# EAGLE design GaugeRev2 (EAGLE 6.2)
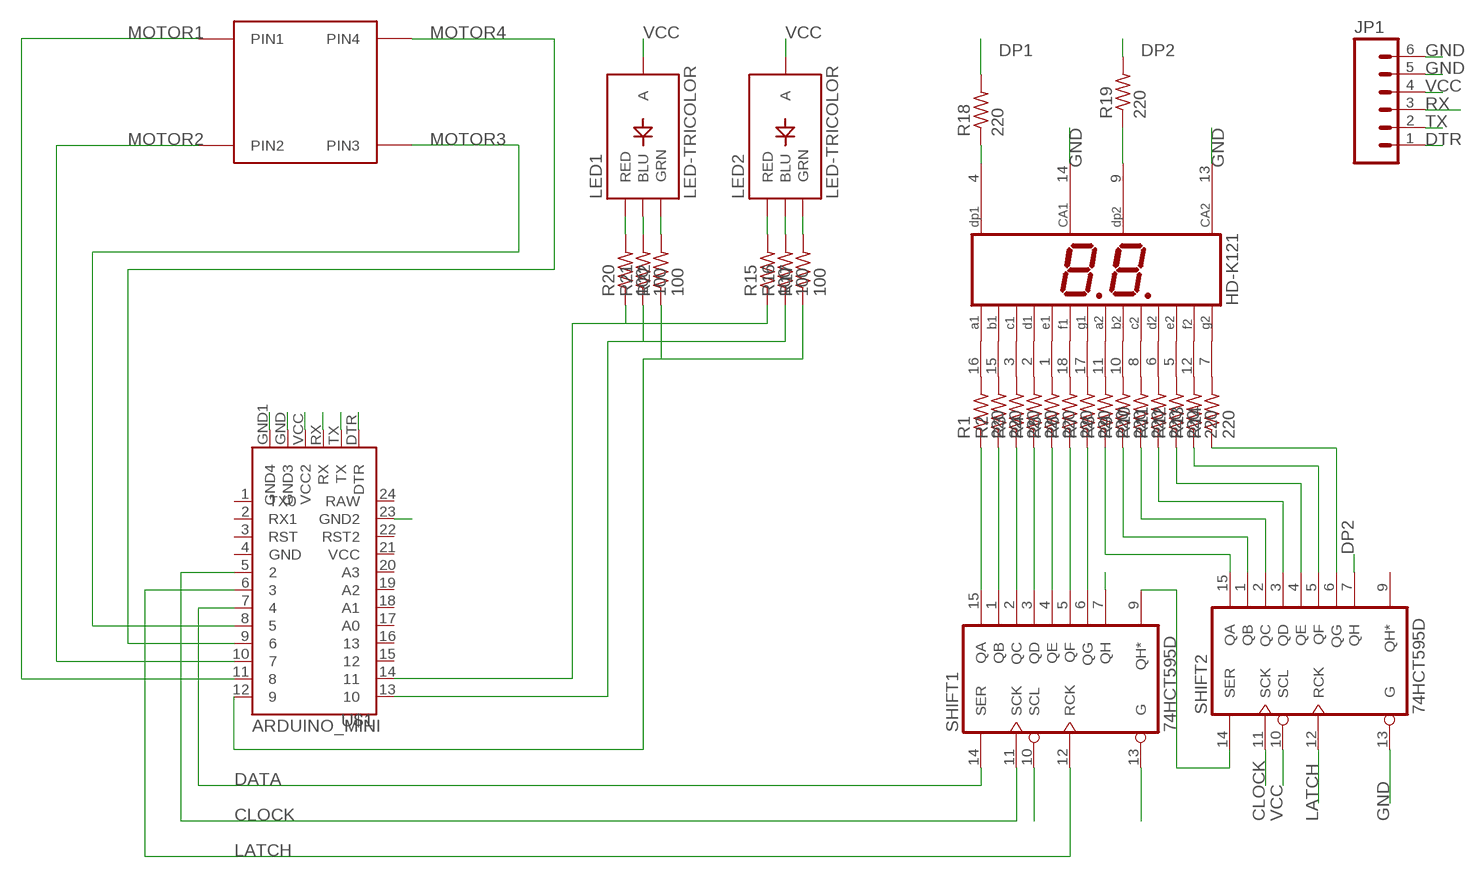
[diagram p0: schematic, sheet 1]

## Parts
DIS2  HD-K121  [HDSP-R]
JP1  M06SIP  [1X06]
LED1  LED-TRICOLOR  [LED-TRICOLOR-SMD]
LED2  LED-TRICOLOR  [LED-TRICOLOR-SMD]
R1  220  R-US_R1206  [R1206]
R2  220  R-US_R1206  [R1206]
R3  220  R-US_R1206  [R1206]
R4  220  R-US_R1206  [R1206]
R5  220  R-US_R1206  [R1206]
R6  220  R-US_R1206  [R1206]
R7  220  R-US_R1206  [R1206]
R8  220  R-US_R1206  [R1206]
R9  220  R-US_R1206  [R1206]
R10  220  R-US_R1206  [R1206]
R11  220  R-US_R1206  [R1206]
R12  220  R-US_R1206  [R1206]
R13  220  R-US_R1206  [R1206]
R14  220  R-US_R1206  [R1206]
R15  100  R-US_R1206  [R1206]
R16  100  R-US_R1206  [R1206]
R17  100  R-US_R1206  [R1206]
R18  220  R-US_R1206  [R1206]
R19  220  R-US_R1206  [R1206]
R20  100  R-US_R1206  [R1206]
R21  100  R-US_R1206  [R1206]
R22  100  R-US_R1206  [R1206]
SHIFT1  74HCT595D  [SO16]
SHIFT2  74HCT595D  [SO16]
U$1  ARDUINO_MINI  [ARDUINO_MINI]
U$4  VID29  [VID29]

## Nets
1: DIS2.4(DP1) R18.1
2: DIS2.9(DP2) R19.1
A1: R1.1 SHIFT1.15(QA)
A2: R8.1 SHIFT2.15(QA)
B1: R2.1 SHIFT1.1(QB)
B2: R9.1 SHIFT2.1(QB)
C1: R3.1 SHIFT1.2(QC)
CLOCK: SHIFT1.11(SCK) SHIFT2.11(SCK) U$1.5
D1: R4.1 SHIFT1.3(QD)
DATA: SHIFT1.14(SER) U$1.7
DP1: R18.2 SHIFT1.7(QH)
DP2: R19.2 SHIFT2.7(QH)
DTR: JP1.1 U$1.DTR
E1: R5.1 SHIFT1.4(QE)
F1: R6.1 SHIFT1.5(QF)
G1: R7.1 SHIFT1.6(QG)
G2: R14.1 SHIFT2.6(QG)
GND: DIS2.13(CA2) DIS2.14(CA1) JP1.5 JP1.6 SHIFT1.13(G) SHIFT2.13(G) U$1.23(GND2) U$1.GND1(GND4) U$1.GND(GND3)
LATCH: SHIFT1.12(RCK) SHIFT2.12(RCK) U$1.6
LED_B: R16.1 R21.1 U$1.13
LED_G: R15.1 R20.1 U$1.14
LED_R: R17.1 R22.1 U$1.12
MOTOR1: U$1.11 U$4.PIN1
MOTOR2: U$1.10 U$4.PIN2
MOTOR3: U$1.8 U$4.PIN3
MOTOR4: U$1.9 U$4.PIN4
N$1: DIS2.16(A1) R1.2
N$2: DIS2.15(B1) R2.2
N$3: DIS2.3(C1) R3.2
N$4: DIS2.2(D1) R4.2
N$5: DIS2.1(E1) R5.2
N$6: DIS2.18(F1) R6.2
N$7: DIS2.17(G1) R7.2
N$8: DIS2.11(A2) R8.2
N$9: DIS2.10(B2) R9.2
N$10: DIS2.8(C2) R10.2
N$11: DIS2.6(D2) R11.2
N$12: DIS2.5(E2) R12.2
N$13: DIS2.12(F2) R13.2
N$14: DIS2.7(G2) R14.2
N$15: LED2.G(GRN) R17.2
N$16: LED2.B(BLU) R16.2
N$19: R10.1 SHIFT2.2(QC)
N$20: R11.1 SHIFT2.3(QD)
N$21: R12.1 SHIFT2.4(QE)
N$22: R13.1 SHIFT2.5(QF)
N$23: LED2.R(RED) R15.2
N$24: LED1.G(GRN) R22.2
N$25: LED1.B(BLU) R21.2
N$26: LED1.R(RED) R20.2
Q*: SHIFT1.9(QH*) SHIFT2.14(SER)
RX: JP1.3 U$1.RX
TX: JP1.2 U$1.TX
VCC: JP1.4 LED1.A LED2.A SHIFT1.10(SCL) SHIFT2.10(SCL) U$1.VCC(VCC2)
Unconnected: SHIFT2.9(QH*) U$1.1(TX0) U$1.2(RX1) U$1.3(RST) U$1.4(GND) U$1.15 U$1.16 U$1.17(A0) U$1.18(A1) U$1.19(A2) U$1.20(A3) U$1.21(VCC) U$1.22(RST2) U$1.24(RAW)

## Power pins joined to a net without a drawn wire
GND: SHIFT1.8(GND) SHIFT2.8(GND)
VCC: SHIFT1.16(VCC) SHIFT2.16(VCC)

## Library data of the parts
DIS2 = HDSP-523E:HD-K121: LED DISPLAY 2 x 1 character 7 segment, decimal points right; OC_FARNELL: unknown; OC_NEWARK: unknown
JP1 = SparkFun:M06: Header 6 Standard 6-pin 0.1" header. Use with straight break away headers (SKU : PRT-00116), right angle break away headers (PRT-00553), swiss pins (PRT-00743), machine pins (PRT-00117), and female headers (PRT-00115). Molex polarized connector foot print use with SKU : PRT-08094 with associated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
LED1 LED2 = SparkFun:LED-TRICOLOR: Tri-Color LED SMD Proven layout and schematic for triple color LED in SMD package - common anode. Spark Fun Electronics SKU : COM-07844
R1-R22 = resistor:R-US_: RESISTOR, American symbol
SHIFT1 SHIFT2 = 74xx-eu:74*595: 8-bit SHIFT REGISTER, output latch
U$1 = SparkFun:ARDUINO_MINI
U$4 = Evans:VID29

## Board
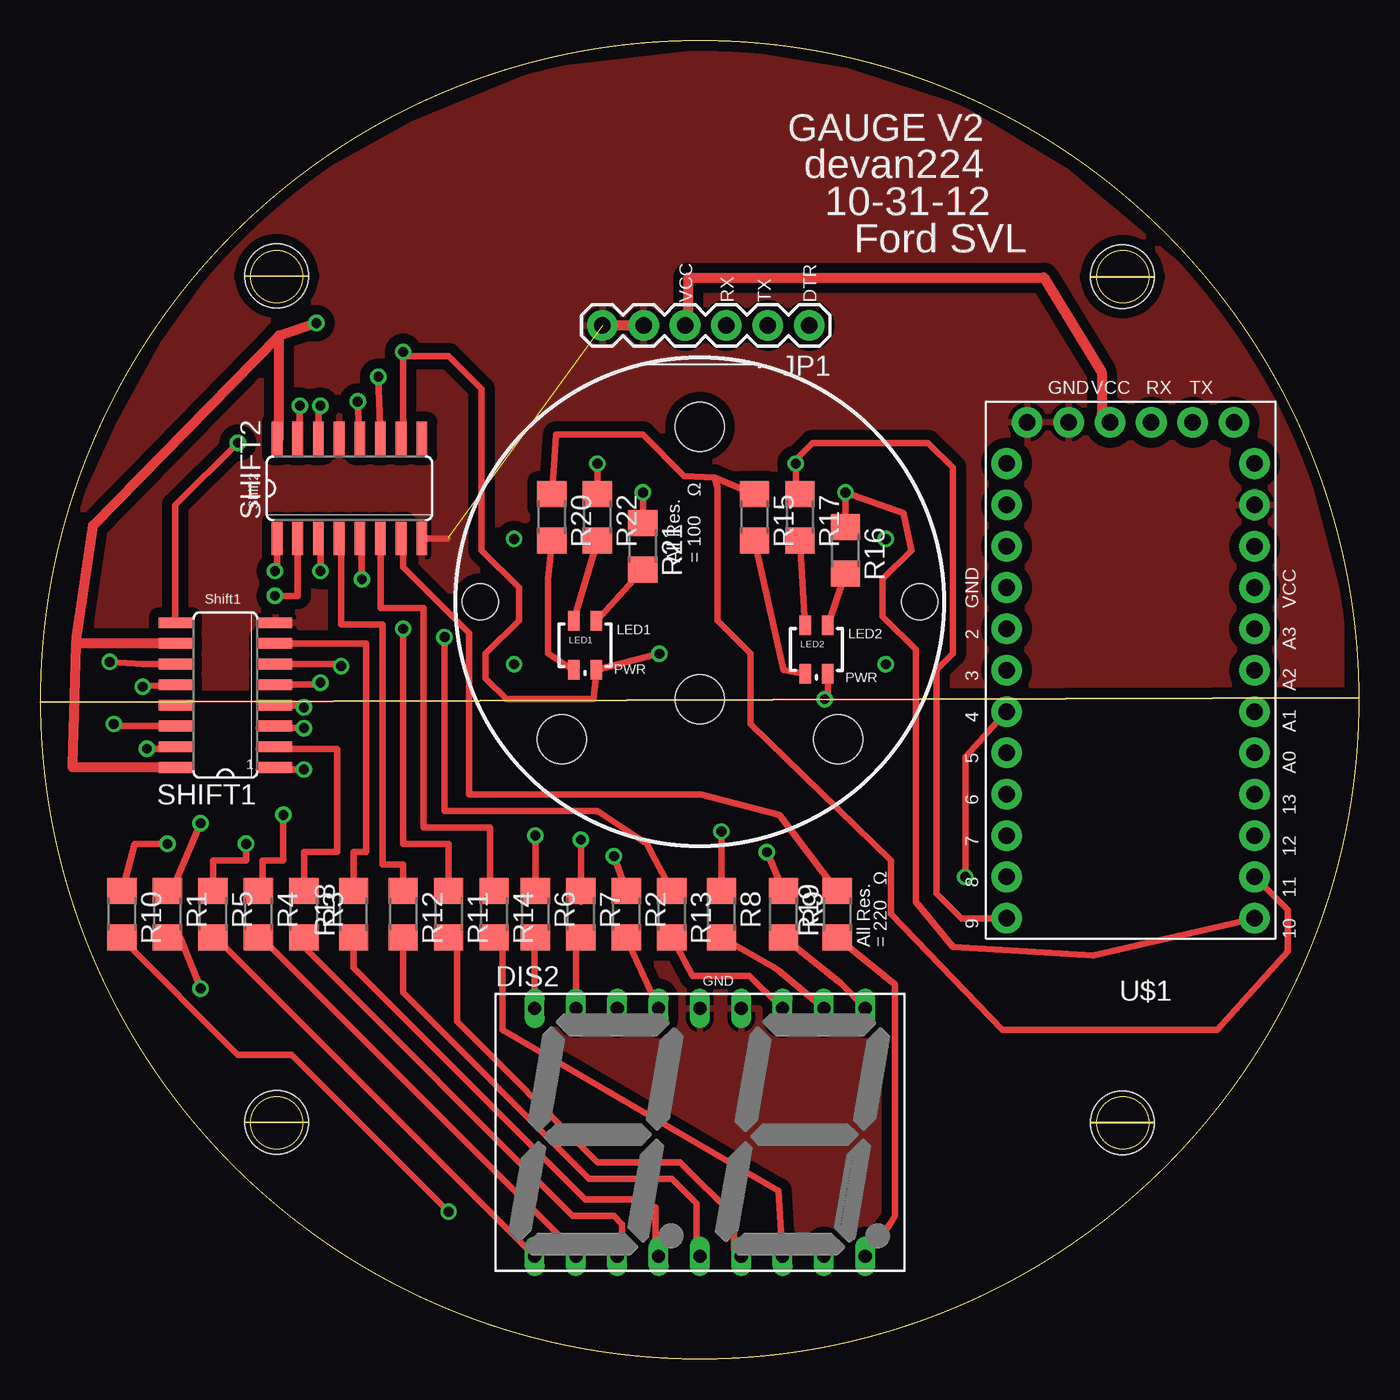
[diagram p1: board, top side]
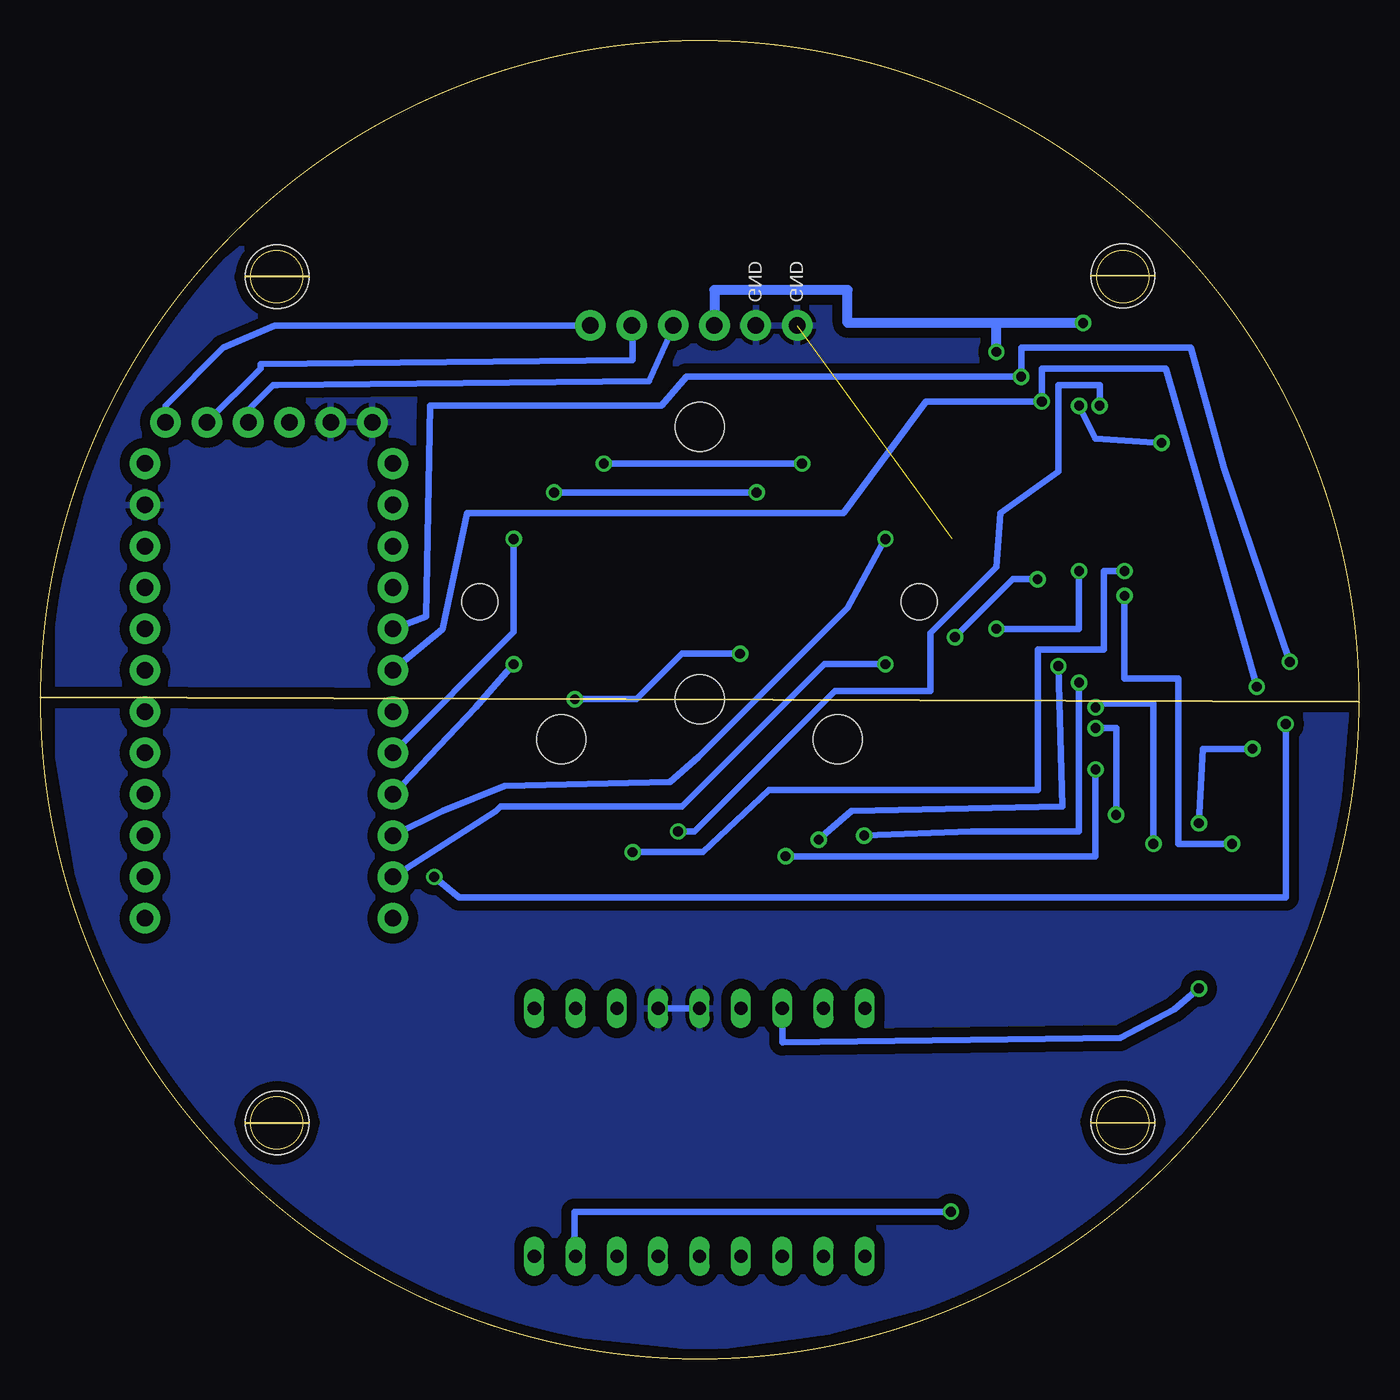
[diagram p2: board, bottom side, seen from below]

Size 81 x 81 mm. Coordinates in mm from the lower left corner, seen from the top.
Outline: circle at 66.5,66.5 radius 1.6
Outline: circle at 14.5,66.5 radius 1.6
Outline: circle at 66.5,14.5 radius 1.6
Outline: circle at 14.5,14.5 radius 1.6
Outline: circle at 40.5,40.5 radius 40.5
Copper layers (1*16): Top 0.0178mm / dielectric 59mil / Bottom 0.0178mm
Design rules: minimum track width 6mil, minimum drill 14mil, track to track 6mil, track to pad 6mil, pad to pad 6mil, via to via 6mil, smd to smd 6mil, copper to edge 20mil, drill to drill 16mil, minimum pad ring 8mil, minimum via ring 8mil, stop-mask expansion 3mil, vias tented up to drill 0mil, thermal gap 10mil
Holes 3.9 mm at 14.5,66.55 66.47,66.5 66.47,14.5 14.5,14.53

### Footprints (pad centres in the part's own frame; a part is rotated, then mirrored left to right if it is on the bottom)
HDSP-R = drill 0.813 long: 1 -10.16,-7.62; 2 -7.62,-7.62; 3 -5.08,-7.62; 4 -2.54,-7.62; 5 0,-7.62; 6 2.54,-7.62; 7 5.08,-7.62; 8 7.62,-7.62; 9 10.16,-7.62; 10 10.16,7.62; 11 7.62,7.62; 12 5.08,7.62; 13 2.54,7.62; 14 0,7.62; 15 -2.54,7.62; 16 -5.08,7.62; 17 -7.62,7.62; 18 -10.16,7.62
1X06 = drill 1.016 pad 1.88: 1 0,0; 2 2.54,0; 3 5.08,0; 4 7.62,0; 5 10.16,0; 6 12.7,0
LED-TRICOLOR-SMD = smd 0.7 x 1.2: A 0.7,-1.5; B 0.7,1.5; G -0.7,1.5; R -0.7,-1.5
R1206 = smd 1.6 x 1.803: 1 -1.422,0; 2 1.422,0
SO16 = smd 0.66 x 2.032: 1 -4.445,-3.073; 2 -3.175,-3.073; 3 -1.905,-3.073; 4 -0.635,-3.073; 5 0.635,-3.073; 6 1.905,-3.073; 7 3.175,-3.073; 8 4.445,-3.073; 9 4.445,3.073; 10 3.175,3.073; 11 1.905,3.073; 12 0.635,3.073; 13 -0.635,3.073; 14 -1.905,3.073; 15 -3.175,3.073; 16 -4.445,3.073
ARDUINO_MINI = drill 1.016 pad 1.88: 1 -7.62,12.7; 2 -7.62,10.16; 3 -7.62,7.62; 4 -7.62,5.08; 5 -7.62,2.54; 6 -7.62,0; 7 -7.62,-2.54; 8 -7.62,-5.08; 9 -7.62,-7.62; 10 -7.62,-10.16; 11 -7.62,-12.7; 12 -7.62,-15.24; 13 7.62,-15.24; 14 7.62,-12.7; 15 7.62,-10.16; 16 7.62,-7.62; 17 7.62,-5.08; 18 7.62,-2.54; 19 7.62,0; 20 7.62,2.54; 21 7.62,5.08; 22 7.62,7.62; 23 7.62,10.16; 24 7.62,12.7; DTR 6.35,15.24; GND -3.81,15.24; GND1 -6.35,15.24; RX 1.27,15.24; TX 3.81,15.24; VCC -1.27,15.24
VID29 = drill 0.6: PIN1 -11.425,-3.85; PIN2 -11.425,3.85; PIN3 11.425,3.85; PIN4 11.425,-3.85 | hole 2.2: 13.5,0; -13.5,0 | hole 3: 0,-6; 0,10.75; -8.5,-8.45; 8.5,-8.45

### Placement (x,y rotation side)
DIS2  40.51,13.92 0 top
JP1  47.22,63.5 180 top
LED1  33.45,43.84 0 top
LED2  47.67,43.58 0 top
R1  7.8,27.33 270 top
R2  35.99,27.33 270 top
R3  16.18,27.33 270 top
R4  13.38,27.33 270 top
R5  10.59,27.33 270 top
R6  30.4,27.33 270 top
R7  33.2,27.33 270 top
R8  41.83,27.33 270 top
R9  45.64,27.33 270 top
R10  5,27.33 270 top
R11  25.07,27.33 270 top
R12  22.27,27.33 270 top
R13  38.78,27.33 270 top
R14  27.86,27.33 270 top
R15  43.86,51.71 270 top
R16  49.45,49.68 270 top
R17  46.66,51.71 270 top
R18  19.23,27.33 90 top
R19  48.94,27.33 90 top
R20  31.42,51.71 270 top
R21  37.01,49.93 270 top
R22  34.21,51.71 270 top
SHIFT1  11.35,40.79 90 top
SHIFT2  18.97,53.49 0 top
U$1  66.98,42.31 0 top
U$4  40.51,46.53 0 top

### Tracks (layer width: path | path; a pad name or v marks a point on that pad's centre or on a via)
1
  Top 0.406: R18.1 19.23,24.03 33.45,9.8 37.01,9.8 37.77,9.29 37.77,6.5 DIS2.4
2
  Top 0.406: R19.1 52.5,23.01 52.5,8.79 52.19,8.28 DIS2.9
A1  (via drill 0.6)
  Top 0.406: R1.1 8.05,28.75 v9.83,32.92 | 7.26,37.49 SHIFT1.15 7.26,37.49 | v6.53,37.49 7.26,37.49
  Bottom 0.406: v9.83,32.92 9.57,37.49 v6.53,37.49
A2  (via drill 0.6)
  Top 0.406: R8.1 v41.83,32.41 | v15.92,58.57 15.92,56.69 SHIFT2.15
  Bottom 0.406: v41.83,32.41 40.82,32.41 37.77,35.46 37.51,35.71 32.18,41.04 26.34,41.04 26.34,44.6 22.27,48.66 22.02,51.97 18.46,54.51 18.46,59.84 15.92,59.84 v15.92,58.57
B1  (via drill 0.6)
  Top 0.406: R2.1 v35.23,30.88 | 13.41,36.22 SHIFT1.1 13.66,36.22 v16.18,36.22
  Bottom 0.406: v35.23,30.88 16.18,30.88 16.18,33.42 v16.18,36.22
B2  (via drill 0.6)
  Top 0.406: R9.1 v44.63,31.14 | v14.4,48.41 14.53,48.41 SHIFT2.1
  Bottom 0.406: v44.63,31.14 40.31,31.14 36.24,34.95 26.85,34.95 19.73,34.95 19.73,43.58 15.67,43.58 15.67,48.41 v14.4,48.41
C1
  Top 0.406: 16.18,37.49 15.67,37.49 | 15.67,37.49 13.41,37.49 SHIFT1.2 | R3.1 16.18,31.14 18.21,31.14 18.21,37.49 15.67,37.49
CLOCK  (via drill 0.6)
  Top 0.406: SHIFT1.11 6.27,42.7 v4.24,42.82 | v20.75,60.35 SHIFT2.11
  Bottom 0.406: v4.24,42.82 8.3,54.76 10.34,62.13 20.75,62.13 v20.75,60.35 41.32,60.35 42.85,58.57 57.07,58.57 57.33,45.62 U$1.5
D1  (via drill 0.6)
  Top 0.406: v16.18,38.76 13.41,38.76 SHIFT1.3 | R4.1 13.64,28.75 13.64,30.63 14.91,30.63 v14.91,33.42
  Bottom 0.406: v14.91,33.42 14.91,38.76 v16.18,38.76
DATA  (via drill 0.6)
  Top 0.406: SHIFT1.14 4.49,38.89 v4.49,39.01 | v56.82,29.61 56.82,36.98 U$1.7
  Bottom 0.406: v4.49,39.01 4.49,28.34 55.29,28.34 v56.82,29.61
DP1
  Top 0.406: SHIFT1.7 19.99,43.97 19.99,31.14 19.23,31.14 R18.2
DP2
  Top 0.406: R19.2 45.39,33.42 40.56,34.69 36.5,34.69 26.34,34.69 | 26.34,34.69 26.34,34.95 | 26.34,34.95 26.34,34.69 | 26.34,34.95 26.34,44.09 26.34,44.6 22.27,48.66 22.27,49.93 22.27,50.29 SHIFT2.7
DTR
  Bottom 0.406: JP1.1 66.62,63.5 69.77,62.13 73.33,58.57 U$1.DTR
E1  (via drill 0.6)
  Top 0.406: SHIFT1.4 15.92,40.16 v16.18,40.03 | R5.1 10.59,30.63 12.62,30.63 v12.62,31.65
  Bottom 0.406: v12.62,31.65 12.62,34.19 12.62,40.28 16.18,40.28 v16.18,40.03
F1  (via drill 0.6)
  Top 0.406: SHIFT1.5 17.07,41.43 v17.19,41.55 | v30.4,32.15 R6.1
  Bottom 0.406: v17.19,41.55 17.19,32.41 23.8,32.41 v30.4,32.15
G1  (via drill 0.6)
  Top 0.406: R7.1 33.2,28.09 R7.1 | SHIFT1.6 18.46,42.7 v18.46,42.57 | v33.2,31.9 33.2,31.39 R7.1
  Bottom 0.406: v18.46,42.57 18.21,33.93 31.16,33.68 v33.2,31.9
G2
  Top 0.406: R14.1 27.61,28.75 27.61,32.66 23.54,32.66 23.54,46.12 20.88,46.12 SHIFT2.6
GND  (1 unrouted)
  Top 0.406: SHIFT2.8 25.01,50.42
  Top 0.61: JP1.5 JP1.6
  Bottom 0.406: DIS2.14 DIS2.13
  pour Bottom (isolate 0.61): 4.75,57.3 7.54,62.38 11.35,67.71 15.92,72.03 22.78,75.84 30.91,79.14 41.83,80.41 49.45,79.14 56.56,76.86 62.91,73.05 70.79,66.44 74.09,61.87 77.39,55.78 79.93,46.12 79.93,36.98 78.41,28.09 76.38,22.76 71.55,15.14 65.71,9.55 58.6,4.72 49.71,1.67 40.05,0.66 32.69,1.67 24.05,3.96 18.97,6.75 15.16,9.55 11.1,13.87 6.27,19.71 3.99,24.53 1.45,32.15 0.68,41.04 1.95,51.2
  pour Top (isolate 0.61): 4.75,57.3 7.54,62.38 11.35,67.71 15.92,72.03 22.78,75.84 30.91,79.14 41.83,80.41 49.45,79.14 56.56,76.86 62.91,73.05 70.79,66.44 74.09,61.87 77.39,55.78 79.93,46.12 79.93,36.98 78.41,28.09 76.38,22.76 71.55,15.14 65.71,9.55 58.6,4.72 49.71,1.67 40.05,0.66 32.69,1.67 24.05,3.96 18.97,6.75 15.16,9.55 11.1,13.87 6.27,19.71 3.99,24.53 1.45,32.15 0.68,41.04 1.95,51.2
LATCH  (via drill 0.6)
  Top 0.406: SHIFT1.12 v6.27,41.3 | v19.48,58.82 SHIFT2.12
  Bottom 0.406: v6.27,41.3 8.56,49.43 11.86,60.86 19.48,60.86 v19.48,58.82 26.59,58.82 31.67,51.97 54.79,51.97 56.31,44.85 U$1.6
LED_B  (via drill 0.6)
  Top 0.406: U$1.13 64.69,24.79 56.06,25.3 53.77,28.09 53.77,39.77 53.77,41.04 53.77,43.58 51.74,45.62 51.74,47.9 53.52,49.68 53.01,51.97 v49.45,53.24 R16.1 | v37.01,53.24 R21.1
  Bottom 0.406: v49.45,53.24 v37.01,53.24
LED_G
  Top 0.406: R20.1 31.67,56.79 37.01,56.79 39.55,54.25 41.41,54.16 | 41.41,54.16 43.61,53.24 R15.1 | U$1.14 76.63,27.58 76.63,25.04 72.31,20.22 59.1,20.22 52.25,27.33 52.25,30.63 43.61,39.01 43.61,43.33 41.58,45.36 41.58,51.97 41.58,53.56 41.41,54.16
LED_R  (via drill 0.6)
  Top 0.406: U$1.12 56.56,27.07 55.04,28.6 55.04,42.31 56.06,43.33 56.06,54.76 54.53,56.28 47.42,56.28 46.4,55.27 | 46.4,55.27 v46.4,55.01 | v46.4,55.01 46.4,53.39 R17.1 | R22.1 v34.21,55.01 | v46.4,55.01 46.4,55.27
  Bottom 0.406: v34.21,55.01 v46.4,55.01
MOTOR1
  Bottom 0.406: U$4.PIN1 32.83,42.68 41.58,33.93 52.75,33.93 53.01,33.68 U$1.11
MOTOR2
  Bottom 0.406: U$4.PIN2 29.13,50.38 31.42,46.12 40.56,36.98 42.34,35.46 52.5,35.2 56.31,33.68 U$1.10
MOTOR3
  Bottom 0.406: U$4.PIN3 51.94,44.66 U$1.8
MOTOR4
  Bottom 0.406: U$4.PIN4 54.28,40.03 U$1.9
N$1  (via drill 0.6)
  Top 0.406: R1.2 8.56,25.91 v9.83,22.76
  Bottom 0.406: v9.83,22.76 11.35,21.49 14.65,19.71 35.43,19.45 DIS2.16
N$2
  Top 0.406: R2.2 36.19,25.4 DIS2.15
N$3
  Top 0.406: R3.2 16.18,25.3 32.69,8.79 35.23,8.79 35.74,8.28 35.74,6.6 DIS2.3
N$4
  Top 0.406: R4.2 13.54,25.91 32.18,7.26 32.18,7.01 DIS2.2
N$5
  Top 0.406: R5.2 10.74,25.91 DIS2.1
N$6
  Top 0.406: R6.2 30.35,25.91 DIS2.18
N$7
  Top 0.406: R7.2 32.89,25.91 DIS2.17
N$8
  Top 0.406: DIS2.11 45.34,23.87 45.13,24.03 R8.2
N$9
  Top 0.406: R9.2 49.15,23.11 DIS2.10
N$10  (via drill 0.6)
  Top 0.406: R10.2 5,25.8 12.11,18.69 15.42,18.69 v25.07,9.04
  Bottom 0.406: v25.07,9.04 48.18,9.04 48.18,6.35 DIS2.8
N$11
  Top 0.406: R11.2 25.58,25.91 25.58,20.72 34.21,12.09 39.29,12.09 42.59,8.79 42.59,6.75 DIS2.6
N$12
  Top 0.406: R12.2 22.27,22.5 33.7,11.07 38.78,11.07 40.31,9.55 40.31,6.5 DIS2.5
N$13
  Top 0.406: DIS2.12 43.56,23.52 40.05,23.52 R13.2
N$14
  Top 0.406: R14.2 28.37,25.91 28.37,20.22 45.34,10.31 DIS2.7
N$15
  Top 0.406: R17.2 LED2.G
N$16
  Top 0.406: R16.2 LED2.B
N$19  (via drill 0.6)
  Top 0.406: R10.1 5.76,31.65 v7.8,31.65 | v14.4,46.89 15.8,46.89 SHIFT2.2
  Bottom 0.406: v14.4,46.89 14.4,41.81 11.1,41.81 11.1,31.65 v7.8,31.65
N$20  (via drill 0.6)
  Top 0.406: R11.1 25.07,30.12 25.07,30.88 25.07,31.65 22.27,31.65 v22.27,44.85 | v17.19,48.41 17.19,50.29 SHIFT2.3
  Bottom 0.406: v17.19,48.41 17.19,44.85 v22.27,44.85
N$21
  Top 0.406: R12.1 22.27,30.38 21,30.38 21,40.28 21,45.11 18.46,45.11 18.46,50.29 SHIFT2.4
N$22  (via drill 0.6)
  Top 0.406: v24.81,44.35 24.81,33.68 34.21,33.68 37.26,31.65 37.77,30.63 R13.1 | v19.73,47.9 19.73,50.29 SHIFT2.5
  Bottom 0.406: v24.81,44.35 21.26,47.9 v19.73,47.9
N$23
  Top 0.406: LED2.R 45.64,42.31 R15.2
N$24
  Top 0.406: R22.2 LED1.G
N$25
  Top 0.406: R21.2 LED1.B
N$26
  Top 0.406: R20.2 31.16,47.9 31.16,43.33 LED1.R
Q*  (via drill 0.6)
  Top 0.406: SHIFT1.9 8.28,52.45 v12.11,56.28 | v17.19,58.57 17.07,58.57 SHIFT2.14
  Bottom 0.406: v12.11,56.28 16.18,56.54 v17.19,58.57
RX
  Bottom 0.406: JP1.3 42.09,63.5 43.61,60.09 66.47,59.84 66.72,59.84 68.5,58.06 68.5,57.81 U$1.RX
TX
  Bottom 0.406: JP1.2 44.63,63.5 44.63,61.36 67.49,61.11 67.49,60.86 U$1.TX
VCC  (via drill 0.6)
  Top 0.406: SHIFT2.16 14.65,56.56 | SHIFT2.10 22.27,56.56 v22.27,61.87 22.53,61.62 25.07,61.62 27.1,59.59 27.1,57.81 27.1,49.68 29.39,47.39 29.39,45.36 27.35,43.33 27.35,41.81 28.62,40.54 33.96,40.54 34.13,41.97 34.13,42.31 | LED2.A 48.37,40.73 v48.18,40.54 | v38.02,43.33 34.13,42.31 | 34.13,42.31 LED1.A
  Top 0.61: SHIFT1.16 3.35,36.35 1.95,36.35 1.95,36.47 2.19,43.86 | 2.19,43.86 2.21,44.35 3.22,51.2 14.65,62.89 | SHIFT1.10 3.22,43.97 2.19,43.97 2.19,43.86 | 14.65,56.56 14.65,62.89 | 14.65,62.89 v16.94,63.65 | JP1.4 39.8,63.5 39.8,66.44 61.64,66.44 65.2,60.6 65.2,58.06 U$1.VCC
  Bottom 0.406: v48.18,40.54 44.37,40.54 41.58,43.33 v38.02,43.33
  Bottom 0.61: v22.27,61.87 22.27,63.65 | 22.27,63.65 31.42,63.65 31.42,65.68 39.6,65.68 JP1.4 | v16.94,63.65 22.27,63.65

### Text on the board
tPlace: GAUGE V2 | devan224 | 10-31-12 | Ford SVL | VCC | RX | TX | DTR | Ω | Shift2 | All Res. | = 100 | Shift1 | LED1 | LED2 | PWR | PWR | 1 | Ω | All Res. | = 220 | GND
bPlace: GND | GND

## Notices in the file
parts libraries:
SparkFun: Licensing: CC v3.0 Share-Alike You are welcome to use this library for commercial purposes.
